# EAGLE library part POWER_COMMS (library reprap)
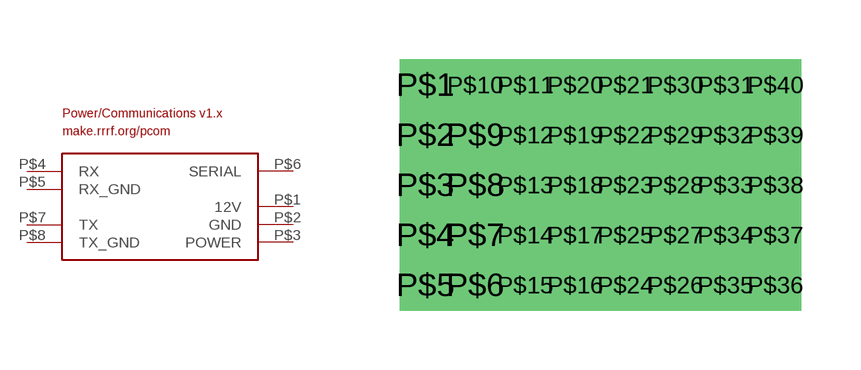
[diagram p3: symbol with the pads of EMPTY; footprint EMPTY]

Designator prefix -

## POWER_COMMS  [EMPTY]
P$1  12V
P$2  GND
P$3  POWER
P$4  RX
P$5  RX_GND
P$6  SERIAL
P$7  TX
P$8  TX_GND

## Footprint EMPTY (pad centres in mm)
drill 0.8 square: P$1 -1.27,5.08; P$2 -1.27,3.81; P$3 -1.27,2.54; P$4 -1.27,1.27; P$5 -1.27,0; P$6 0,0; P$7 0,1.27; P$8 0,2.54; P$9 0,3.81; P$10 0,5.08; P$11 1.27,5.08; P$12 1.27,3.81; P$13 1.27,2.54; P$14 1.27,1.27; P$15 1.27,0; P$16 2.54,0; P$17 2.54,1.27; P$18 2.54,2.54; P$19 2.54,3.81; P$20 2.54,5.08; P$21 3.81,5.08; P$22 3.81,3.81; P$23 3.81,2.54; P$24 3.81,0; P$25 3.81,1.27; P$26 5.08,0; P$27 5.08,1.27; P$28 5.08,2.54; P$29 5.08,3.81; P$30 5.08,5.08; P$31 6.35,5.08; P$32 6.35,3.81; P$33 6.35,2.54; P$34 6.35,1.27; P$35 6.35,0; P$36 7.62,0; P$37 7.62,1.27; P$38 7.62,2.54; P$39 7.62,3.81; P$40 7.62,5.08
